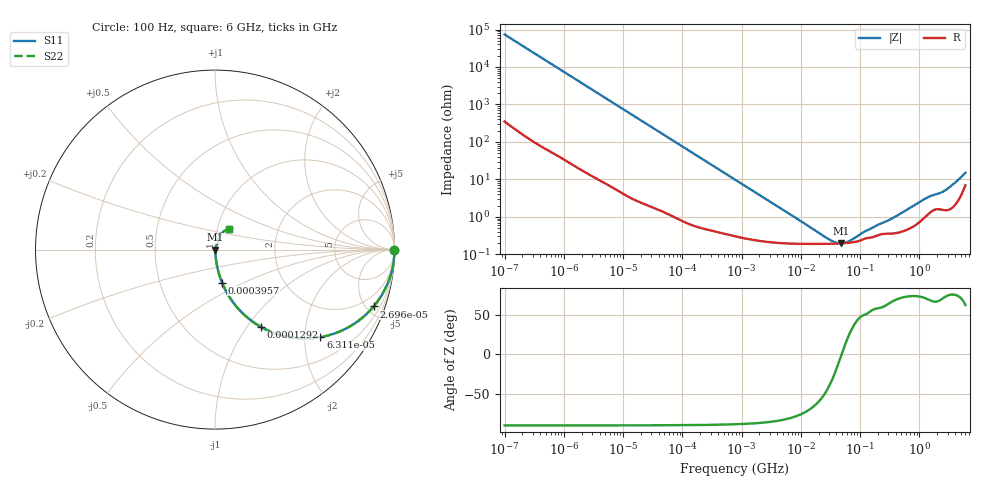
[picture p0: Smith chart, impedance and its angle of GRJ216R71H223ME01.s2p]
!Murata Part Number: GRJ216R71H223ME01
!These Parameters are Measured in Series Mode Connection
!Data Generated on Jun 19, 2026
!  o--ll--o
!Port1  Port2
!  o------o
!Operation Temp=25[degC], DC Bias Voltage=0[V]
!Freq. Start=100[Hz] Stop=6[GHz] 401[Steps]
# Hz S RI R 50
!Freq.(Hz) S11(Real) S11(Imag) S21(Real) S21(Imag) S12(Real) S12(Imag) S22(Real) S22(Imag)
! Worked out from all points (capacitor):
!   401 points, 100 Hz to 6 GHz, reference 50 ohm
!   read as one part in series: C = 21.5 nF near 109 Hz
!   lowest |Z| = 196 mohm at 47.65 MHz (marker M1)
!   series resonance near 48.74 MHz, so ESL is about 500 pH
!   S11 on the Smith chart (normalised r, x): 100 Hz: open; 26.96 kHz: 1.04, -5.57; 63.12 kHz: 1.02, -2.39; 129.2 kHz: 1.01, -1.17; 395.7 kHz: 1.01, -0.38; 6 GHz: 1.14, +0.27
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100  1 -0.00135  8.2e-06 0.00135  8.2e-06 0.00135  1 -0.00135
2008  0.9991 -0.0269  0.000852 0.0269  0.000852 0.0269  0.9991 -0.0269
8801  0.9858 -0.1158  0.0142 0.1158  0.0142 0.1158  0.9858 -0.1158
16473  0.9529 -0.209  0.0471 0.209  0.0471 0.209  0.9529 -0.209
26957  0.8842 -0.3164  0.1158 0.3164  0.1158 0.3164  0.8842 -0.3164
40335  0.7751 -0.4135  0.2249 0.4135  0.2249 0.4135  0.7751 -0.4135
63115  0.5876 -0.4877  0.4124 0.4877  0.4124 0.4877  0.5876 -0.4877
90302  0.4129 -0.4874  0.5871 0.4874  0.5871 0.4874  0.4129 -0.4874
129199  0.258 -0.4321  0.742 0.4321  0.742 0.4321  0.258 -0.4321
211427  0.1175 -0.3151  0.8825 0.3151  0.8825 0.3151  0.1175 -0.3151
395726  0.0392 -0.1842  0.9608 0.1842  0.9608 0.1842  0.0392 -0.1842
774597  0.0126 -0.0973  0.9874 0.0973  0.9874 0.0973  0.0126 -0.0973
2481164  0.00313 -0.0309  0.9969 0.0309  0.9969 0.0309  0.00313 -0.0309
1.555665e7  0.00191 -0.00448  0.9981 0.00448  0.9981 0.00448  0.00191 -0.00448
3.184506e7  0.00191 -0.0014  0.9981 0.0014  0.9981 0.0014  0.00191 -0.0014
4.764863e7  0.00195 -7.15e-05  0.998 7.15e-05  0.998 7.15e-05  0.00195 -7.15e-05
6.518806e7  0.00203 0.000938  0.998 -0.000938  0.998 -0.000938  0.00203 0.000938
1.166697e8  0.00257 0.00303  0.9974 -0.00303  0.9974 -0.00303  0.00257 0.00303
3.124326e8  0.00358 0.00745  0.9964 -0.00745  0.9964 -0.00745  0.00358 0.00745
1.251881e9  0.0105 0.0282  0.9895 -0.0282  0.9895 -0.0282  0.0105 0.0282
2.562649e9  0.0169 0.044  0.9831 -0.044  0.9831 -0.044  0.0169 0.044
6e9  0.0793 0.1144  0.9207 -0.1144  0.9207 -0.1144  0.0793 0.1144
